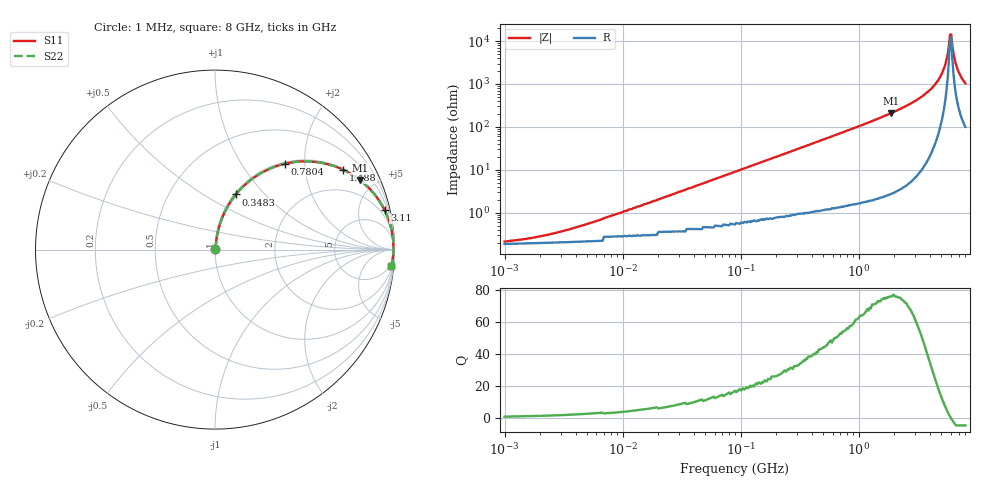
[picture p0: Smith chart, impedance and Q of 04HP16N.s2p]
# MHz S MA R 50
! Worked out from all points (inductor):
!   391 points, 1 MHz to 8 GHz, reference 50 ohm
!   read as one part in series: L = 16 nH near 6.771 MHz
!   highest Q = 76.1 at 1.873 GHz (marker M1), where L = 17.7 nH
!   self-resonance near 5.929 GHz
!   S11 on the Smith chart (normalised r, x): 1 MHz: 1.00, +0.00; 348.3 MHz: 1.02, +0.70; 780.4 MHz: 1.03, +1.59; 1.488 GHz: 1.04, +3.19; 3.11 GHz: 1.15, +8.55; 8 GHz: 3, -21
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1  0.002015 29.8  0.998 -0.1  0.998 -0.1  0.002015 29.8
2.091  0.002862 47.0  0.998 -0.1  0.998 -0.1  0.002862 47.0
4.576  0.005115 63.5  0.998 -0.3  0.998 -0.3  0.005115 63.5
20.466  0.021 79.6  0.996 -1.2  0.996 -1.2  0.021 79.6
89.443  0.089 81.4  0.991 -5.1  0.991 -5.1  0.089 81.4
348.347  0.329 69.2  0.935 -19.2  0.935 -19.2  0.329 69.2
409.325  0.379 66.3  0.916 -22.3  0.916 -22.3  0.379 66.3
780.351  0.618 50.8  0.775 -38.2  0.775 -38.2  0.618 50.8
1487.687  0.842 31.9  0.528 -57.3  0.528 -57.3  0.842 31.9
1830.556  0.892 26.1  0.44 -63.2  0.44 -63.2  0.892 26.1
1873.229  0.897 25.5  0.43 -63.8  0.43 -63.8  0.897 25.5
3110.034  0.97 13.1  0.227 -75.9  0.227 -75.9  0.97 13.1
4196.316  0.989 6.9  0.12 -81.2  0.12 -81.2  0.989 6.9
5045.817  0.994 3.3  0.058 -82.0  0.058 -82.0  0.994 3.3
5406.987  0.994 2.0  0.035 -79.6  0.035 -79.6  0.994 2.0
5662.017  0.994 1.1  0.02 -73.1  0.02 -73.1  0.994 1.1
5929.076  0.994 0.2  0.007006 -34.3  0.007006 -34.3  0.994 0.2
6067.292  0.994 -0.2  0.006978 31.0  0.006978 31.0  0.994 -0.2
6353.467  0.993 -1.1  0.02 70.2  0.02 70.2  0.993 -1.1
6653.139  0.993 -1.9  0.035 76.6  0.035 76.6  0.993 -1.9
7295.554  0.99 -3.7  0.065 79.3  0.065 79.3  0.99 -3.7
8000  0.986 -5.5  0.096 79.0  0.096 79.0  0.986 -5.5
